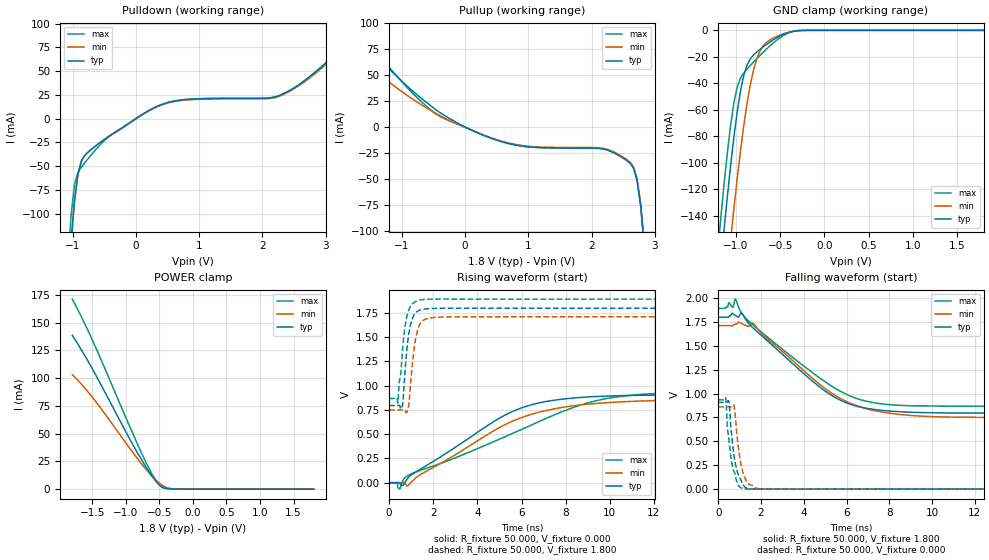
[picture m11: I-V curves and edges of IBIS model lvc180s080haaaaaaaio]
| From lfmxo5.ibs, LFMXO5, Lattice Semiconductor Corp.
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[Model] lvc180s080haaaaaaaio
Model_type I/O
Polarity   Non-Inverting
Enable   Active-Low
Vinl =  0.630V
Vinh =  1.170V
Vmeas =  0.900V
Cref =  0.0F
Rref =  1.000M
Vref =  0.0V
C_comp   5.000pF   4.000pF   5.500pF
[Temperature Range]   25.000   0.125k   -40.000
[Voltage Range]   1.800V   1.710V   1.890V
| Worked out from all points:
|   slope of the pulldown table from 0 to 0.27 V, typ, clamps not added: 25.1 ohm
|   slope of the pullup table from 0 to 0.27 V, typ, clamps not added: 36.8 ohm
|   GND clamp passes 1 mA (typ) near -0.37 V on its own axis
|   POWER clamp passes 1 mA (typ) near -0.42 V on its own axis
|   rising waveform, R_fixture 50.000, V_fixture 0.000: 20-80 % time 3.79ns typ, 4.1ns min, 5.83ns max; typ from 0 V to 0.908 V
|   rising waveform, R_fixture 50.000, V_fixture 1.800: 20-80 % time 267ps typ, 286ps min, 290ps max; typ from 0.796 V to 1.8 V
|   falling waveform, R_fixture 50.000, V_fixture 1.800: 20-80 % time 3.13ns typ, 3.18ns min, 3.55ns max; typ from 1.8 V to 0.796 V
|   falling waveform, R_fixture 50.000, V_fixture 0.000: 20-80 % time 324ps typ, 330ps min, 330ps max; typ from 0.908 V to 0 V
[GND_clamp]
|Voltage   I(typ)   I(min)   I(max)
-1.8V     -665.5mA   -701.9mA   -644.7mA
-1.208V   -203.2mA   -259.3mA   -168.6mA
-1.171V   -176.5mA   -233.3mA   -141.8mA
-1.134V   -150.7mA   -207.7mA   -116.3mA
-1.06V    -102.3mA   -158.3mA   -71.8mA
-1.023V   -80.78mA   -134.8mA   -54.83mA
-986mV    -61.78mA   -112.4mA   -42.93mA
-875mV    -26.33mA   -55.53mA   -29.29mA
-764mV    -16.38mA   -21.41mA   -21.4mA
-616mV    -8.858mA   -7.288mA   -11.79mA
-283mV    -142.7uA   -287uA     -113.6uA
1.8V      0A         0A         0A
[POWER_clamp]
|Voltage   I(typ)   I(min)   I(max)
-1.8V     138.7mA    103.3mA    171.3mA
-1.678V   127mA      95.65mA    157.2mA
-1.53V    111.7mA    85.11mA    138.4mA
-1.345V   91.17mA    70.52mA    113.2mA
-938mV    44.71mA    36.47mA    55.67mA
-753mV    25.22mA    21.78mA    30.82mA
-605mV    11.26mA    11.4mA     13.08mA
-494mV    3.49mA     5.157mA    3.227mA
-457mV    1.898mA    3.519mA    1.512mA
-383mV    542.5uA    1.315mA    536.2uA
-235mV    73.61uA    152.3uA    57.83uA
1.8V      0A         0A         0A
[Pulldown]
|Voltage   I(typ)   I(min)   I(max)
-1.8V     -1.123A    -1.123A    -1.379A
-1.085V   -187mA     -187mA     -163mA
-1.03V    -131.9mA   -131.9mA   -104mA
-975mV    -88.04mA   -88.04mA   -69.67mA
-920mV    -59.22mA   -59.22mA   -56.86mA
-810mV    -38.63mA   -38.63mA   -46.55mA
-425mV    -18.55mA   -18.55mA   -18.85mA
180mV     7.522mA    7.296mA    7.522mA
730mV     19.66mA    19.07mA    19.66mA
2.27V     24.3mA     23.57mA    24.3mA
2.765V    45.03mA    43.68mA    45.03mA
3.6V      96.4mA     93.5mA     96.4mA
[Pullup]
|Voltage   I(typ)   I(min)   I(max)
-1.8V     92.7mA     71.09mA    101.5mA
-1.735V   88.8mA     68.19mA    96.8mA
-855mV    36.27mA    28.13mA    34.32mA
-415mV    14.75mA    11.73mA    11.05mA
135mV     -3.78mA    -3.666mA   -3.78mA
740mV     -16.47mA   -15.97mA   -16.47mA
2.115V    -20.5mA    -19.88mA   -20.5mA
2.335V    -24.14mA   -23.41mA   -24.14mA
2.665V    -39.44mA   -38.25mA   -39.44mA
2.72V     -51.1mA    -49.57mA   -51.1mA
2.83V     -110.7mA   -107.4mA   -110.7mA
3.6V      -932.5mA   -904.6mA   -932.5mA
[Ramp]
| variable   typ   min   max
dV/dt_r   0.545/3.795n   0.512/4.120n   0.560/5.831n
dV/dt_f   0.602/3.125n   0.576/3.181n   0.614/3.556n
R_load = 50.000
[Rising Waveform]
R_fixture = 50.000
V_fixture = 0.000
V_fixture_min = 0.000
V_fixture_max = 0.000
|  time   V(typ)   V(min)   V(max)
0s        66.63uV    -485.3uV   428.6uV
355ps     61.52uV    -758.3uV   2.171mV
480ps     -1.914mV   -506.2uV   -66.96mV
634ps     -28.46mV   -249.5uV   27.42mV
824ps     40.97mV    -33.58mV   69.27mV
5.1ns     678.2mV    580.4mV    458.9mV
7.01ns    832.7mV    738.6mV    652.5mV
9.034ns   884.1mV    809.9mV    824.6mV
11.06ns   900.2mV    839mV      904mV
20ns      908.2mV    861.1mV    934.4mV
[Rising Waveform]
R_fixture = 50.000
V_fixture = 1.800
V_fixture_min = 1.710
V_fixture_max = 1.890
|  time   V(typ)   V(min)   V(max)
0s        796mV      750.1mV    868.6mV
393ps     796.1mV    749.7mV    822mV
600ps     792.6mV    750.3mV    1.349V
704ps     1.1V       751.2mV    1.586V
844ps     1.462V     751.5mV    1.75V
904ps     1.555V     826.2mV    1.79V
1.145ns   1.736V     1.405V     1.861V
1.384ns   1.779V     1.629V     1.883V
2.474ns   1.8V       1.708V     1.894V
20ns      1.8V       1.712V     1.892V
[Falling Waveform]
R_fixture = 50.000
V_fixture = 1.800
V_fixture_min = 1.710
V_fixture_max = 1.890
|  time   V(typ)   V(min)   V(max)
0s        1.8V       1.712V     1.892V
495ps     1.808V     1.712V     1.953V
685ps     1.837V     1.712V     1.903V
804ps     1.818V     1.726V     1.99V
1.107ns   1.841V     1.731V     1.839V
1.657ns   1.682V     1.732V     1.713V
4.985ns   1.029V     1.056V     1.126V
6.927ns   846.6mV    841.9mV    920.3mV
10ns      799.4mV    759.3mV    870mV
20ns      796mV      750.1mV    868.6mV
[Falling Waveform]
R_fixture = 50.000
V_fixture = 0.000
V_fixture_min = 0.000
V_fixture_max = 0.000
|  time   V(typ)   V(min)   V(max)
0s        908.2mV    861.1mV    934.4mV
349ps     907.9mV    860.9mV    956.2mV
434ps     915.9mV    860.9mV    639.5mV
493ps     919.7mV    860.9mV    536.3mV
733ps     359.7mV    877.2mV    188.4mV
974ps     132.8mV    388.5mV    30.77mV
1.173ns   42.03mV    162.1mV    4.979mV
1.415ns   5.455mV    56.42mV    51.32uV
1.972ns   39.8uV     2.083mV    -551.5uV
20ns      66.63uV    -485.3uV   428.6uV
